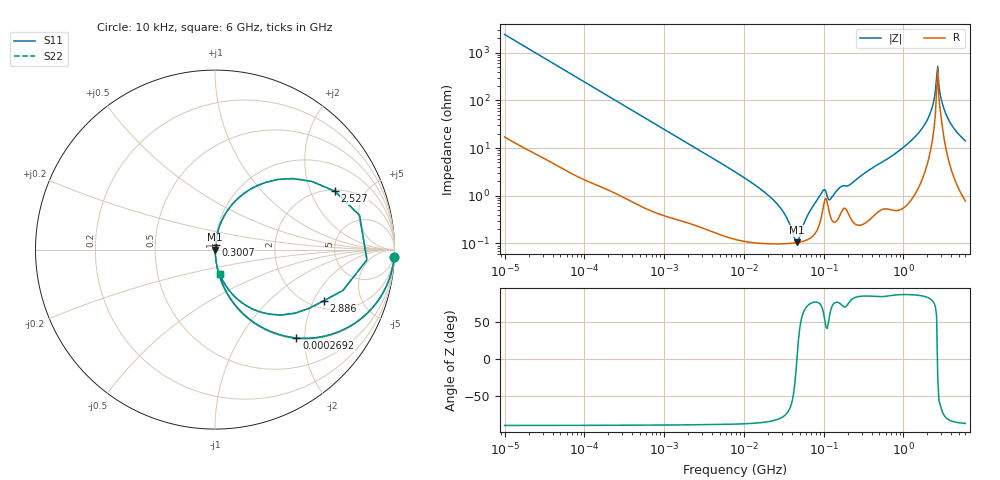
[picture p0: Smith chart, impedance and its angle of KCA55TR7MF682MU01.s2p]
!Murata Part Number: KCA55TR7MF682MU01
!These Parameters are Measured in Series Mode Connection
!Data Generated on Jan 08, 2026
!  o--ll--o
!Port1  Port2
!  o------o
!Operation Temp=25[degC], DC Bias Voltage=0[V]
!Freq. Start=10[kHz] Stop=6[GHz] 401[Steps]
# Hz S RI R 50
!Freq.(Hz) S11(Real) S11(Imag) S21(Real) S21(Imag) S12(Real) S12(Imag) S22(Real) S22(Imag)
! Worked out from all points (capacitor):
!   401 points, 10 kHz to 6 GHz, reference 50 ohm
!   read as one part in series: C = 6.6 nF near 10.69 kHz
!   lowest |Z| = 105 mohm at 46.68 MHz (marker M1)
!   series resonance near 46.26 MHz, so ESL is about 1.8 nH
!   S11 on the Smith chart (normalised r, x): 10 kHz: 1, -48; 269.2 kHz: 1.02, -1.82; 300.7 MHz: 1.00, +0.05; 2.527 GHz: 2.07, +3.01; 2.886 GHz: 2.33, -2.41; 6 GHz: 1.02, -0.28
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10000  0.998 -0.0414  0.00201 0.0414  0.00201 0.0414  0.998 -0.0414
92862  0.8707 -0.3312  0.1293 0.3312  0.1293 0.3312  0.8707 -0.3312
269211  0.4534 -0.4922  0.5466 0.4922  0.5466 0.4922  0.4534 -0.4922
862344  0.0789 -0.2624  0.9211 0.2624  0.9211 0.2624  0.0789 -0.2624
7745967  0.00221 -0.0316  0.9978 0.0316  0.9978 0.0316  0.00221 -0.0316
2.565129e7  0.00102 -0.00687  0.999 0.00687  0.999 0.00687  0.00102 -0.00687
3.347128e7  0.000997 -0.00365  0.999 0.00365  0.999 0.00365  0.000997 -0.00365
4.667948e7  0.00104 0.000103  0.999 -0.000103  0.999 -0.000103  0.00104 0.000103
7.193098e7  0.00141 0.0055  0.9986 -0.0055  0.9986 -0.0055  0.00141 0.0055
9.70341e7  0.00484 0.0113  0.9952 -0.0113  0.9952 -0.0113  0.00484 0.0113
1.224735e8  0.00362 0.00772  0.9964 -0.00772  0.9964 -0.00772  0.00362 0.00772
1.598104e8  0.00402 0.0142  0.996 -0.0142  0.996 -0.0142  0.00402 0.0142
3.006542e8  0.00315 0.0266  0.9968 -0.0266  0.9968 -0.0266  0.00315 0.0266
6.67969e8  0.00898 0.0617  0.991 -0.0617  0.991 -0.0617  0.00898 0.0617
1.811831e9  0.0997 0.2563  0.9003 -0.2563  0.9003 -0.2563  0.0997 0.2563
2.286837e9  0.3497 0.3907  0.6503 -0.3907  0.6503 -0.3907  0.3497 0.3907
2.526803e9  0.6678 0.3252  0.3322 -0.3252  0.3322 -0.3252  0.6678 0.3252
2.700612e9  0.8464 -0.0574  0.1536 0.0574  0.1536 0.0574  0.8464 -0.0574
2.886376e9  0.6059 -0.2854  0.3941 0.2854  0.3941 0.2854  0.6059 -0.2854
3.189254e9  0.3696 -0.3643  0.6304 0.3643  0.6304 0.3643  0.3696 -0.3643
3.766309e9  0.149 -0.2953  0.851 0.2953  0.851 0.2953  0.149 -0.2953
6e9  0.0268 -0.1363  0.9732 0.1363  0.9732 0.1363  0.0268 -0.1363
